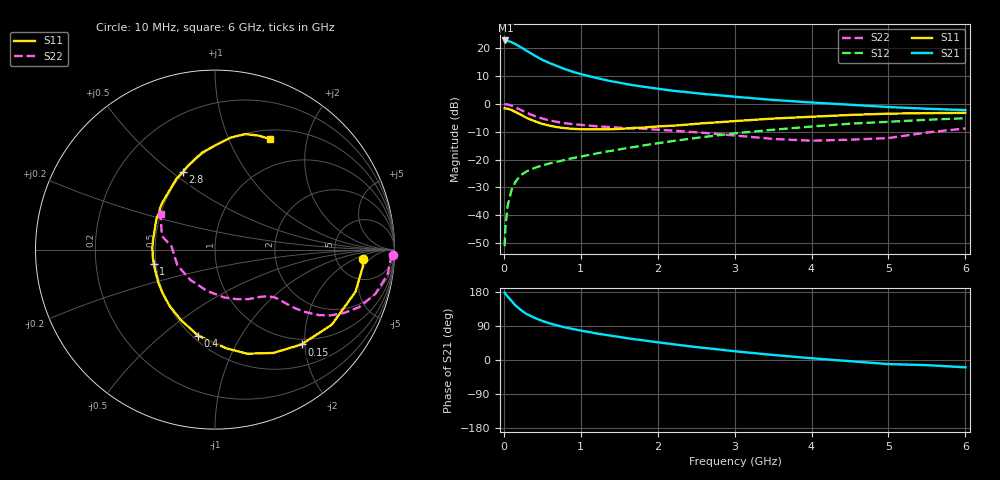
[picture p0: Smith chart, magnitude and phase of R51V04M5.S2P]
! SIEMENS Small Signal Semiconductors
! BFR183
! Si NPN RF Bipolar Junction Transistor in SOT23
! VCE = 1 V  IC = 4.5 mA
! Common Emitter S-Parameters:  May  1996
# GHz  S  MA  R  50
!  f  S11  S21  S12  S22
! GHz  MAG  ANG  MAG  ANG  MAG  ANG  MAG  ANG
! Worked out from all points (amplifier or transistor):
!   36 points, 10 MHz to 6 GHz, reference 50 ohm
!   highest |S21| = 22.7 dB at 20 MHz (marker M1)
!   |S21| within 3 dB of that: start of sweep to 255 MHz
!   unconditionally stable (mu >= 1): 1.024 GHz to 2.865 GHz
!   at 250 MHz: K = 0.40, MSG = 22.4 dB, |S12| = -25.0 dB
!   at 1.4 GHz: K = 1.08, MAG = 10.7 dB, |S12| = -16.9 dB
!   at 6 GHz: K = 0.93, MSG = 1.5 dB, |S12| = -5.2 dB
!   S11 on the Smith chart (normalised r, x): 10 MHz: 10, -3; 150 MHz: 0.89, -1.93; 400 MHz: 0.53, -0.67; 1 GHz: 0.49, -0.09; 2.8 GHz: 0.50, +0.55; 6 GHz: 0.61, +1.43
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0.01  0.8279 -3.6  13.55 177.7  0.0028 86.9  0.9898 -1.6
0.02  0.8285 -6.8  13.67 174.8  0.006 87.7  0.9797 -3.3
0.05  0.8173 -16.7  13.38 167.4  0.015 80.9  0.9717 -8.2
0.1  0.7737 -32.7  12.76 155.8  0.0286 73.3  0.9266 -15.5
0.15  0.7152 -47.6  11.78 144.3  0.0399 67.0  0.8642 -21.8
0.2  0.6616 -60.5  10.77 135.5  0.0487 62.0  0.8017 -26.1
0.25  0.6071 -72.8  9.775 127.5  0.0561 58.0  0.7399 -29.7
0.3  0.5548 -83.2  8.851 121.0  0.0618 55.9  0.6853 -32.2
0.4  0.4884 -101.1  7.318 111.4  0.0709 52.3  0.6031 -35.0
0.5  0.4368 -115.5  6.14 103.1  0.0785 51.1  0.5447 -36.4
0.6  0.4035 -128.8  5.338 96.4  0.0858 51.0  0.5019 -37.1
0.7  0.3799 -140.2  4.702 90.8  0.0918 51.6  0.4715 -37.6
0.8  0.3652 -149.9  4.159 86.0  0.0991 51.6  0.4479 -38.1
1  0.3507 -167.0  3.416 77.7  0.1131 52.6  0.4193 -39.1
1.1  0.3488 -174.4  3.151 74.0  0.1205 53.2  0.4075 -40.2
1.6  0.3619 155.9  2.25 57.6  0.1607 54.2  0.3659 -45.9
2.2  0.4053 131.7  1.714 41.6  0.215 52.2  0.3309 -56.6
2.8  0.4675 112.6  1.421 27.7  0.2741 47.5  0.2855 -72.3
3.5  0.5438 97.8  1.173 13.3  0.3424 39.6  0.2345 -100.8
4.5  0.631 81.9  0.963 -3.1  0.44 27.1  0.2271 -157.5
5.5  0.68 69.0  0.815 -13.6  0.5173 14.7  0.3057 165.6
6  0.6882 63.5  0.772 -19.3  0.5512 6.7  0.3619 147.0
